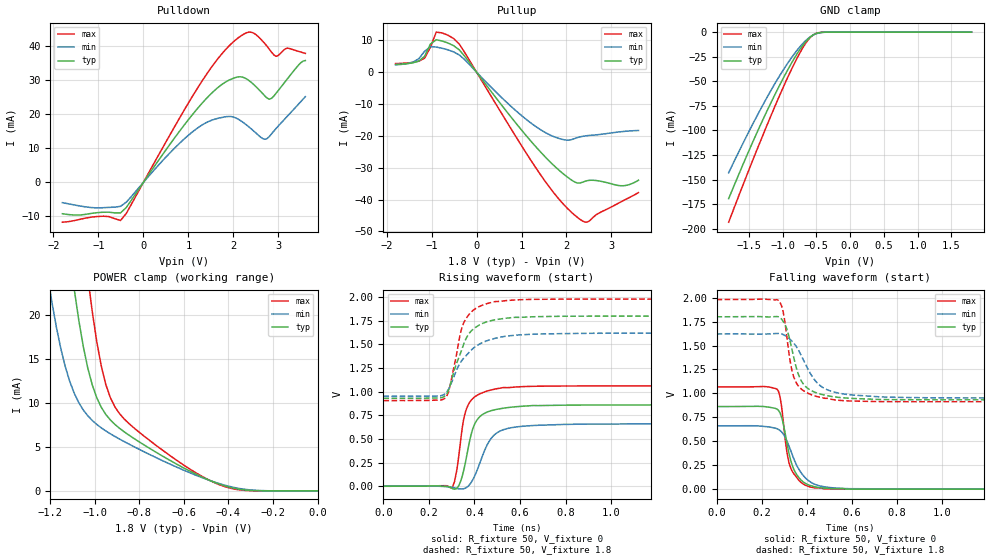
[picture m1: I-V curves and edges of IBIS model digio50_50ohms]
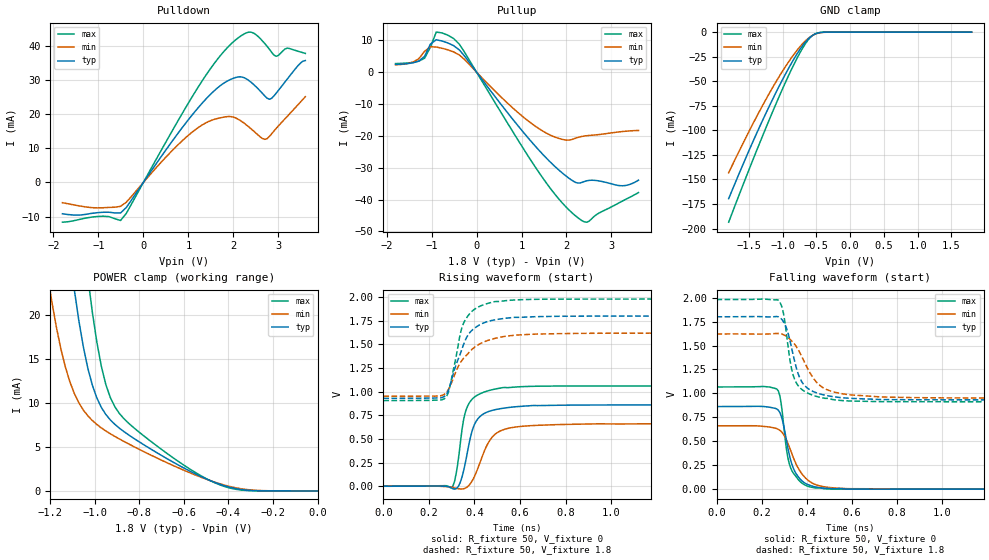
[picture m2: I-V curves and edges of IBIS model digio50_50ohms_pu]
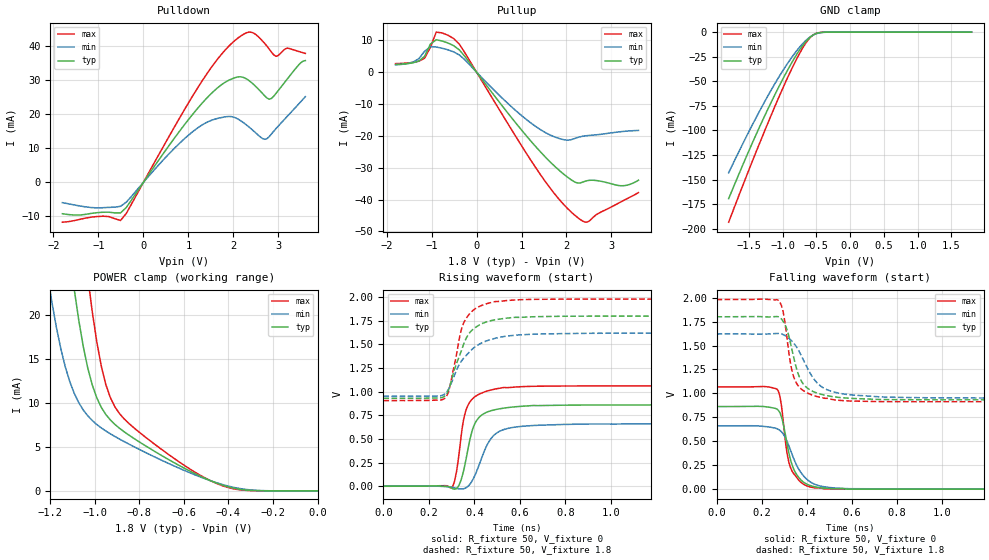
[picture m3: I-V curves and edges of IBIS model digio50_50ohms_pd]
[IBIS ver]   4.0
[File name]   tusb1210.ibs
[File rev]   1.0
[Date]   Thu Nov 25 16:58:20 2010
[Source]   Texas Instruments Incorporated.
   Analog-eLab, HPA
   12500 TI Blvd
   Dallas, TX -75243
   For Support e-mail: elab_ibis@list.ti.com
[Notes] Reision History: 1.0
- Combined Pulldown/Pull up for dn_ls, dn_hs, dn_fs, dp_ls, dp_hs,dp_fs reflects
  the behavior based on simulations.
- GND Clamp value of digio50_50ohms_pu never becomming zero reflects
  the behavior based on simulations.
- POWER Clamp value of digio50_50ohms_pd never becomming zero reflects
  the behavior based on simulations.
[Disclaimer]
 This product is designed as an aid for customers of Texas Instruments.
 No warranties, either expressed or implied, with respect to this third
 party software (if any) or with respect to its fitness for any
 particular purpose is claimed by Texas Instruments or the author. The
 software (if any) is provided solely on an "as is" basis. The entire
 risk as to its quality and performance is with the customer
[Copyright] (C) Copyright 2010 Texas Instruments Incorporated.
   All rights reserved.
|   COMPONENT: TUSB1210
[Component]   TUSB1210
[Manufacturer]   Texas Instruments.
[Package]
|   typ   min   max
R_pkg   6.77e-02  1.30e-03  1.34e-01
L_pkg   1.06e-09  1.42e-10  1.98e-09
C_pkg   1.51e-13  8.64e-14  2.16e-13
[Pin] signal_name   model_name  R_pin   L_pin   C_pin
1   REFCLK   in50_vio_rst0	 1.34e-01  1.98e-09  2.08e-13
2   NXT   digio50_50ohms_ppud 1.17e-01  1.71e-09  2.12e-13
3   DATA0   digio50_50ohms_ppud 1.08e-01  1.56e-09  1.99e-13
4   DATA1   digio50_50ohms_ppud 1.03e-01  1.49e-09  1.93e-13
5   DATA2   digio50_50ohms_ppud 1.03e-01  1.49e-09  1.97e-13
6   DATA3   digio50_50ohms_ppud 1.07e-01  1.56e-09  2.05e-13
7   DATA4   digio50_50ohms_ppud 1.14e-01  1.67e-09  2.05e-13
9   DATA5   digio50_50ohms_ppud 1.30e-03  1.48e-10  8.64e-14
10   DATA6   digio50_50ohms_ppud 1.27e-01  1.87e-09  1.95e-13
11   CS   in50_vio_rst0	 1.08e-01  1.56e-09  1.97e-13
12   NC   NC   1.04e-01  1.50e-09  1.95e-13
13   DATA7   digio50_50ohms_ppud 1.12e-01  1.63e-09  2.03e-13
14   REFSEL2   in50_vio_rst1	 1.13e-01  1.64e-09  2.01e-13
17   CPEN   digout_od_os_3p1	 1.11e-01  1.60e-09  1.95e-13
18   DP   dp   1.30e-03  1.42e-10  1.02e-13
19   DM   dn   1.30e-03  1.48e-10  8.64e-14
20   VDD33   Power		 1.32e-01  1.94e-09  1.99e-13
21   VBAT   Power		 1.23e-01  1.80e-09  2.16e-13
22   VBUS   Power		 1.15e-01  1.67e-09  2.15e-13
23   ID   NC   1.08e-01  1.55e-09  1.99e-13
26   CLOCK   digio50_50ohms_ppud 1.04e-01  1.50e-09  1.91e-13
27   RESETB   in50_vio_rst0	 1.04e-01  1.49e-09  1.90e-13
28   VDD18_1   Power		 1.12e-01  1.62e-09  1.95e-13
29   STP   digio50_50ohms_ppud 1.30e-03  1.48e-10  8.64e-14
30   VDD18_2   Power		 1.30e-03  1.48e-10  8.64e-14
31   DIR   digio50_50ohms_ppud 1.14e-01  1.66e-09  2.01e-13
32   VDDIO   Power		 1.05e-01  1.52e-09  1.95e-13
| Remark: If you runnin LS and FS simulation in differential Rx mode,
|   please uncomment "For LS and FS simulation" line.
|   While for HS Simulation in differential Rx mode,
|   uncomment "For HS simulation only" line. Please do take note only
|   one line can be sitch on for specific simulation.
[Diff Pin] inv_pin vdiff tdelay_typ tdelay_min tdelay_max
|18 19   0.200V   NA   NA   NA   |For LS/FS simulation only
18 19   0.150V   NA   NA   NA   |For HS simulation only
[Model Selector]   digio50_50ohms_ppud
digio50_50ohms   Pullup-down disabled
digio50_50ohms_pu   Pullup enabled
digio50_50ohms_pd   Pulldown enabled
[Model Selector]   digout_od_os_3p1
digout_od_3p1   Open-drain mode
digout_os_3p1   Open-source mode
digout_cmos_3p1   CMOS mode
[Model Selector]   out50_bat
out50_bat_cmos   Output buffer under VBAT NMOS/PMOS enabled
out50_bat_nmos   Output buffer under VBAT NMOS enabled
out50_bat_pmos   Output buffer under VBAT PMOS enabled
[Model Selector]  dp
dp_fs   Full-Speed mode
dp_hs   High-Speed mode
dp_ls   Low-Speed mode
[Model Selector]  dn
dn_fs   Full-Speed mode
dn_hs   High-Speed mode
dn_ls   Low-Speed mode
| Models and submodels in the file (17): digio50_50ohms (I/O), digio50_50ohms_pu (I/O), digio50_50ohms_pd (I/O), in50_vio_rst0 (Input), in50_vio_rst1 (Input), out50_bat_cmos (Output), out50_bat_nmos (Open_drain), out50_bat_pmos (Open_source), dp_fs (I/O), dp_hs (I/O), dp_ls (I/O), dn_fs (I/O), dn_hs (I/O), dn_ls (I/O), digout_cmos_3p1 (Output), digout_od_3p1 (Open_drain), digout_os_3p1 (Open_source)
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|   Model: digio50_50ohms
|   Description:  I/O buffer for ULPI buffer PU/PD disabled
[Model]   digio50_50ohms
Model_type   I/O
Polarity   Non-Inverting
Enable   Active-Low
Vinh =   1.667
Vinl =   1.364
Vmeas =   0.900
Vref =   0
Cref =   5e-12
Rref =   100e3
|variable   typ   min   max
C_comp   1.086p   1.040p   1.121p
[Model Spec]
|Thresholds   typ   min   max
Vinh+   1.667   1.500   1.833
Vinh-   1.364   1.227   1.500
Vinl+   1.667   1.500   1.833
Vinl-   1.364   1.227   1.500
[Temperature Range]   27   125   -40
[Voltage Range]   1.8   1.62   1.98
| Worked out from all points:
|   slope of the pulldown table from 0 to 0.27 V, typ, clamps not added: 51.8 ohm
|   slope of the pullup table from 0 to 0.27 V, typ, clamps not added: 53.2 ohm
|   GND clamp passes 1 mA (typ) near -0.48 V on its own axis
|   POWER clamp passes 1 mA (typ) near -0.47 V on its own axis
|   rising waveform, R_fixture 50, V_fixture 0: 20-80 % time 54.8ps typ, 76.2ps min, 45.4ps max; typ from 0 V to 0.86 V
|   rising waveform, R_fixture 50, V_fixture 1.8: 20-80 % time 82.7ps typ, 112ps min, 63.2ps max; typ from 0.931 V to 1.8 V
|   falling waveform, R_fixture 50, V_fixture 0: 20-80 % time 55.1ps typ, 81.7ps min, 41.4ps max; typ from 0.863 V to 0 V
|   falling waveform, R_fixture 50, V_fixture 1.8: 20-80 % time 65ps typ, 103ps min, 48.7ps max; typ from 1.8 V to 0.932 V
[GND Clamp]
| digio50_50ohms
|Voltage   I(typ)   I(min)   I(max)
-1.8V     -169.5mA   -143.1mA   -193.4mA
-1.598V   -136.3mA   -114.5mA   -157.3mA
-1.395V   -104.5mA   -87.3mA    -122.2mA
-1.193V   -74.69mA   -61.74mA   -88.34mA
-1.032V   -52.26mA   -42.95mA   -62.34mA
-869.7mV  -31.66mA   -26.14mA   -38mA
-748.3mV  -18.08mA   -15.27mA   -21.59mA
-627mV    -7.357mA   -6.7mA     -8.334mA
-546.1mV  -2.821mA   -2.927mA   -2.841mA
-465.2mV  -709.6uA   -933.8uA   -580uA
-303.4mV  -9.124uA   -34.65uA   -2.526uA
1.8V      19.41nA    6.754uA    15.04nA
[POWER Clamp]
| digio50_50ohms
|Voltage   I(typ)   I(min)   I(max)
-1.8V     230mA      184.4mA    260.1mA
-1.214V   50.81mA    24.76mA    72.72mA
-1.193V   45.55mA    21.5mA     66.74mA
-1.153V   35.62mA    16.15mA    55.07mA
-1.092V   22.81mA    11.06mA    38.57mA
-1.032V   13.92mA    8.517mA    24.25mA
-1.011V   12mA       7.982mA    20.28mA
-991mV    10.55mA    7.534mA    16.89mA
-930.3mV  8.051mA    6.48mA     10.58mA
-829.2mV  6.029mA    5.081mA    7.251mA
-424.7mV  636.6uA    708.5uA    557.6uA
0V        19.41nA    47.88nA    41nA
[Pulldown]
| digio50_50ohms
|Voltage   I(typ)   I(min)   I(max)
-1.8V     -9.222mA   -5.96mA    -11.7mA
-895.8mV  -8.773mA   -7.446mA   -9.946mA
-508.3mV  -8.983mA   -7.037mA   -11.2mA
1.2V      21.68mA    15.95mA    27.64mA
1.8V      29.29mA    19.23mA    38.64mA
2.15V     31.05mA    18.24mA    42.9mA
2.45V     28.8mA     15.11mA    43.89mA
2.65V     26.12mA    12.89mA    41.53mA
2.8V      24.46mA    13.51mA    39.15mA
2.95V     26.21mA    15.86mA    37.06mA
3.2V      30.42mA    19.45mA    39.49mA
3.6V      35.82mA    25.21mA    37.92mA
[Pullup]
| digio50_50ohms
|Voltage   I(typ)   I(min)   I(max)
-1.8V     2.414mA    2.279mA    2.667mA
-1.413V   2.907mA    3.119mA    3.042mA
-1.154V   4.963mA    6.516mA    4.36mA
-1.025V   8.782mA    7.956mA    7.803mA
-895.8mV  10.15mA    7.861mA    12.55mA
-508.3mV  8.286mA    6.333mA    10.52mA
1.4V      -24.71mA   -17.87mA   -31.75mA
1.95V     -32.18mA   -21.25mA   -41.74mA
2.35V     -34.6mA    -20.18mA   -46.68mA
2.5V      -33.98mA   -19.9mA    -46.81mA
3.25V     -35.67mA   -18.66mA   -40.43mA
3.6V      -33.93mA   -18.33mA   -37.83mA
[Ramp]
| digio50_50ohms
|variable   typ   min   max
dV/dt_r   0.863/5.506e-11   0.661/7.618e-11   1.068/4.610e-11
dV/dt_f   0.870/6.539e-11   0.669/1.029e-10   1.074/4.951e-11
R_load =   50
[Rising Waveform]
| digio50_50ohms
R_fixture =   50
V_fixture =   0
V_fixture_min =   0
V_fixture_max =   0
|Time   V(typ)   V(min)   V(max)
0s        348.4uV    407.9uV    39.07nV
303.5ps   -25.21mV   -11.62mV   -7.697mV
321.2ps   -23.49mV   -23.4mV    153.7mV
341.4ps   67.66mV    -28.79mV   526.8mV
356.6ps   210mV      -23.23mV   751.6mV
381.4ps   507.3mV    25.8mV     896.4mV
414.2ps   710.8mV    185.8mV    965.6mV
480.6ps   804mV      527.1mV    1.023V
604.6ps   845.1mV    632.9mV    1.053V
9.107ns   860.3mV    661.1mV    1.062V
[Rising Waveform]
| digio50_50ohms
R_fixture =   50
V_fixture =   1.8
V_fixture_min =   1.62
V_fixture_max =   1.98
|Time   V(typ)   V(min)   V(max)
0s        930.6mV    951.8mV    906.4mV
268ps     950.3mV    973.3mV    926mV
285.7ps   1.014V     1.024V     994.6mV
294.6ps   1.081V     1.067V     1.082V
312.3ps   1.237V     1.175V     1.287V
341.4ps   1.426V     1.319V     1.648V
370.8ps   1.596V     1.401V     1.8V
445.2ps   1.732V     1.53V      1.924V
586.9ps   1.787V     1.599V     1.972V
9.107ns   1.8V       1.62V      1.98V
[Falling Waveform]
| digio50_50ohms
R_fixture =   50
V_fixture =   0
V_fixture_min =   0
V_fixture_max =   0
|Time   V(typ)   V(min)   V(max)
0s        862.7mV    661.7mV    1.067V
267.2ps   837.3mV    631.9mV    1.046V
281.1ps   798.7mV    614mV      971.1mV
295.9ps   682.3mV    575mV      707.6mV
311.7ps   487.1mV    504mV      392.5mV
333.3ps   266.7mV    374.7mV    197.4mV
358.7ps   141.4mV    234.5mV    111.7mV
398.7ps   54.93mV    107.4mV    36.34mV
488.6ps   8.651mV    21.17mV    2.83mV
10.37ns   31.52uV    30.23uV    11.42uV
[Falling Waveform]
| digio50_50ohms
R_fixture =   50
V_fixture =   1.8
V_fixture_min =   1.62
V_fixture_max =   1.98
|Time   V(typ)   V(min)   V(max)
0s        1.8V       1.621V     1.98V
274.2ps   1.8V       1.625V     1.973V
295.9ps   1.751V     1.614V     1.846V
311.7ps   1.671V     1.592V     1.591V
333.3ps   1.471V     1.548V     1.251V
361.8ps   1.207V     1.458V     1.081V
394ps     1.073V     1.306V     1.016V
454ps     997.5mV    1.092V     961.6mV
592.3ps   948.2mV    984.8mV    920.5mV
10.37ns   932.4mV    951.5mV    912.2mV
|   Model: digio50_50ohms_pu
|   Description:  I/O buffer for ULPI buffer PU enabled
[Model]   digio50_50ohms_pu
Model_type   I/O
Polarity   Non-Inverting
Enable   Active-Low
Vinh =   1.667
Vinl =   1.364
Vmeas =   0.900
Vref =   0
Cref =   5e-12
Rref =   100e3
|variable   typ   min   max
C_comp   1.086p   1.040p   1.121p
[Model Spec]
|Thresholds   typ   min   max
Vinh+   1.667   1.500   1.833
Vinh-   1.364   1.227   1.500
Vinl+   1.667   1.500   1.833
Vinl-   1.364   1.227   1.500
[Temperature Range]   27   125   -40
[Voltage Range]   1.8   1.62   1.98
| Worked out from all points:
|   slope of the pulldown table from 0 to 0.27 V, typ, clamps not added: 51.8 ohm
|   slope of the pullup table from 0 to 0.27 V, typ, clamps not added: 53.3 ohm
|   GND clamp passes 1 mA (typ) near -0.48 V on its own axis
|   POWER clamp passes 1 mA (typ) near -0.46 V on its own axis
|   rising waveform, R_fixture 50, V_fixture 0: 20-80 % time 54.8ps typ, 76.2ps min, 45.4ps max; typ from 0 V to 0.86 V
|   rising waveform, R_fixture 50, V_fixture 1.8: 20-80 % time 82.7ps typ, 112ps min, 63.2ps max; typ from 0.931 V to 1.8 V
|   falling waveform, R_fixture 50, V_fixture 0: 20-80 % time 55.1ps typ, 81.7ps min, 41.4ps max; typ from 0.863 V to 0 V
|   falling waveform, R_fixture 50, V_fixture 1.8: 20-80 % time 65ps typ, 103ps min, 48.7ps max; typ from 1.8 V to 0.932 V
[GND Clamp]
| digio50_50ohms_pu
|Voltage   I(typ)   I(min)   I(max)
-1.8V     -169.5mA   -143.1mA   -193.5mA
-1.598V   -136.3mA   -114.6mA   -157.3mA
-1.395V   -104.6mA   -87.32mA   -122.3mA
-1.193V   -74.72mA   -61.76mA   -88.37mA
-1.032V   -52.29mA   -42.97mA   -62.37mA
-869.7mV  -31.68mA   -26.16mA   -38.03mA
-748.3mV  -18.1mA    -15.28mA   -21.62mA
-627mV    -7.378mA   -6.717mA   -8.361mA
-546.1mV  -2.842mA   -2.944mA   -2.868mA
-465.2mV  -730.7uA   -950.8uA   -606.8uA
-303.4mV  -29.85uA   -51.32uA   -28.89uA
1.8V      19.33nA    7.928uA    -2.076uA
[POWER Clamp]
| digio50_50ohms_pu
|Voltage   I(typ)   I(min)   I(max)
-1.8V     230mA      184.4mA    260.1mA
-1.214V   50.81mA    24.76mA    72.72mA
-1.193V   45.55mA    21.5mA     66.74mA
-1.153V   35.62mA    16.15mA    55.07mA
-1.092V   22.81mA    11.06mA    38.57mA
-1.032V   13.92mA    8.519mA    24.25mA
-1.011V   12mA       7.984mA    20.29mA
-991mV    10.55mA    7.536mA    16.89mA
-930.3mV  8.053mA    6.482mA    10.58mA
-829.2mV  6.032mA    5.083mA    7.254mA
-424.7mV  638.9uA    710.2uA    560.6uA
0V        19.33nA    47.31nA    40.57nA
[Pulldown]
| digio50_50ohms_pu
|Voltage   I(typ)   I(min)   I(max)
-1.8V     -9.196mA   -5.938mA   -11.67mA
-895.8mV  -8.751mA   -7.428mA   -9.918mA
-508.3mV  -8.962mA   -7.02mA    -11.17mA
1.2V      21.68mA    15.95mA    27.65mA
1.8V      29.29mA    19.23mA    38.65mA
2.15V     31.05mA    18.23mA    42.9mA
2.45V     28.79mA    15.11mA    43.88mA
2.65V     26.12mA    12.89mA    41.52mA
2.8V      24.46mA    13.5mA     39.14mA
2.95V     26.2mA     15.86mA    37.06mA
3.2V      30.42mA    19.45mA    39.49mA
3.6V      35.82mA    25.21mA    37.92mA
[Pullup]
| digio50_50ohms_pu
|Voltage   I(typ)   I(min)   I(max)
-1.8V     2.413mA    2.278mA    2.666mA
-1.413V   2.906mA    3.118mA    3.042mA
-1.154V   4.962mA    6.515mA    4.359mA
-1.025V   8.78mA     7.954mA    7.801mA
-895.8mV  10.15mA    7.859mA    12.55mA
-508.3mV  8.284mA    6.332mA    10.52mA
1.4V      -24.69mA   -17.86mA   -31.73mA
1.95V     -32.16mA   -21.24mA   -41.72mA
2.35V     -34.57mA   -20.16mA   -46.65mA
2.5V      -33.96mA   -19.88mA   -46.78mA
3.25V     -35.65mA   -18.63mA   -40.4mA
3.6V      -33.9mA    -18.31mA   -37.8mA
[Ramp]
| digio50_50ohms_pu
|variable   typ   min   max
dV/dt_r   0.863/5.506e-11   0.661/7.618e-11   1.068/4.610e-11
dV/dt_f   0.870/6.539e-11   0.669/1.029e-10   1.074/4.951e-11
R_load =   50
[Rising Waveform]
| digio50_50ohms_pu
R_fixture =   50
V_fixture =   0
V_fixture_min =   0
V_fixture_max =   0
|Time   V(typ)   V(min)   V(max)
0s        348.5uV    407.9uV    39.08nV
303.5ps   -25.3mV    -11.66mV   -7.449mV
321.2ps   -23.38mV   -23.43mV   154.7mV
336.4ps   34.32mV    -28.24mV   425.4mV
351.6ps   156.8mV    -26.57mV   696.2mV
374.4ps   427.1mV    5.616mV    869.1mV
418.6ps   723.7mV    213.9mV    971.3mV
471.8ps   798.1mV    501.1mV    1.018V
524.9ps   824.7mV    596.3mV    1.044V
7.289ns   860.3mV    661.1mV    1.062V
[Rising Waveform]
| digio50_50ohms_pu
R_fixture =   50
V_fixture =   1.8
V_fixture_min =   1.62
V_fixture_max =   1.98
|Time   V(typ)   V(min)   V(max)
0s        930.6mV    951.8mV    906.4mV
268.1ps   950.5mV    973.5mV    926.2mV
285.8ps   1.015V     1.024V     995.2mV
294.7ps   1.082V     1.068V     1.083V
312.4ps   1.238V     1.175V     1.288V
341.5ps   1.426V     1.319V     1.649V
367.3ps   1.581V     1.392V     1.788V
439.3ps   1.726V     1.524V     1.919V
569.2ps   1.786V     1.595V     1.969V
7.289ns   1.8V       1.62V      1.98V
[Falling Waveform]
| digio50_50ohms_pu
R_fixture =   50
V_fixture =   0
V_fixture_min =   0
V_fixture_max =   0
|Time   V(typ)   V(min)   V(max)
0s        862.7mV    661.7mV    1.067V
267.2ps   837.4mV    632mV      1.046V
281ps     799.2mV    614.2mV    972.1mV
295.8ps   683.3mV    575.3mV    709.5mV
311.6ps   488.2mV    504.4mV    393.7mV
333.2ps   267.2mV    375.1mV    197.7mV
358.6ps   141.6mV    234.8mV    111.9mV
398.6ps   54.98mV    107.5mV    36.37mV
488.6ps   8.649mV    21.16mV    2.828mV
10.37ns   31.5uV     30.21uV    11.41uV
[Falling Waveform]
| digio50_50ohms_pu
R_fixture =   50
V_fixture =   1.8
V_fixture_min =   1.62
V_fixture_max =   1.98
|Time   V(typ)   V(min)   V(max)
0s        1.8V       1.621V     1.98V
274.1ps   1.8V       1.625V     1.973V
295.8ps   1.752V     1.614V     1.847V
311.6ps   1.672V     1.593V     1.593V
333.2ps   1.472V     1.548V     1.252V
361.7ps   1.207V     1.458V     1.081V
394ps     1.073V     1.306V     1.016V
454ps     997.5mV    1.092V     961.6mV
592.4ps   948.2mV    984.8mV    920.4mV
10.37ns   932.4mV    951.5mV    912.2mV
|   Model: digio50_50ohms_pd
|   Description:  I/O buffer for ULPI buffer PD enabled
[Model]   digio50_50ohms_pd
Model_type   I/O
Polarity   Non-Inverting
Enable   Active-Low
Vinh =   1.667
Vinl =   1.364
Vmeas =   0.900
Vref =   0
Cref =   5e-12
Rref =   100e3
|variable   typ   min   max
C_comp   1.086p   1.040p   1.121p
[Model Spec]
|Thresholds   typ   min   max
Vinh+   1.667   1.500   1.833
Vinh-   1.364   1.227   1.500
Vinl+   1.667   1.500   1.833
Vinl-   1.364   1.227   1.500
[Temperature Range]   27   125   -40
[Voltage Range]   1.8   1.62   1.98
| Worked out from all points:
|   slope of the pulldown table from 0 to 0.27 V, typ, clamps not added: 51.8 ohm
|   slope of the pullup table from 0 to 0.27 V, typ, clamps not added: 53.3 ohm
|   GND clamp passes 1 mA (typ) near -0.48 V on its own axis
|   POWER clamp passes 1 mA (typ) near -0.46 V on its own axis
|   rising waveform, R_fixture 50, V_fixture 0: 20-80 % time 54.8ps typ, 76.2ps min, 45.4ps max; typ from 0 V to 0.86 V
|   rising waveform, R_fixture 50, V_fixture 1.8: 20-80 % time 82.7ps typ, 112ps min, 63.2ps max; typ from 0.931 V to 1.8 V
|   falling waveform, R_fixture 50, V_fixture 0: 20-80 % time 55.1ps typ, 81.7ps min, 41.4ps max; typ from 0.863 V to 0 V
|   falling waveform, R_fixture 50, V_fixture 1.8: 20-80 % time 65ps typ, 103ps min, 48.7ps max; typ from 1.8 V to 0.932 V
[GND Clamp]
| digio50_50ohms_pd
|Voltage   I(typ)   I(min)   I(max)
-1.8V     -169.5mA   -143.1mA   -193.4mA
-1.598V   -136.3mA   -114.6mA   -157.3mA
-1.395V   -104.5mA   -87.3mA    -122.2mA
-1.193V   -74.69mA   -61.74mA   -88.35mA
-1.032V   -52.27mA   -42.95mA   -62.34mA
-869.7mV  -31.66mA   -26.14mA   -38mA
-748.3mV  -18.09mA   -15.27mA   -21.6mA
-627mV    -7.36mA    -6.702mA   -8.338mA
-546.1mV  -2.824mA   -2.929mA   -2.845mA
-465.2mV  -712.7uA   -936.2uA   -583.8uA
-303.4mV  -11.86uA   -36.83uA   -5.896uA
1.8V      18.01uA    22.42uA    20.92uA
[POWER Clamp]
| digio50_50ohms_pd
|Voltage   I(typ)   I(min)   I(max)
-1.8V     230mA      184.4mA    260.2mA
-1.214V   50.83mA    24.78mA    72.75mA
-1.193V   45.58mA    21.52mA    66.77mA
-1.153V   35.64mA    16.17mA    55.09mA
-1.092V   22.84mA    11.07mA    38.6mA
-1.032V   13.94mA    8.534mA    24.28mA
-1.011V   12.02mA    7.999mA    20.31mA
-991mV    10.57mA    7.551mA    16.91mA
-930.3mV  8.072mA    6.496mA    10.61mA
-829.2mV  6.05mA     5.098mA    7.277mA
-424.7mV  656.8uA    724.7uA    583.6uA
0V        18.01uA    14.54uA    23.03uA
[Pulldown]
| digio50_50ohms_pd
|Voltage   I(typ)   I(min)   I(max)
-1.8V     -9.22mA    -5.958mA   -11.7mA
-895.8mV  -8.77mA    -7.444mA   -9.943mA
-508.3mV  -8.98mA    -7.035mA   -11.2mA
1.2V      21.66mA    15.94mA    27.63mA
1.8V      29.27mA    19.22mA    38.62mA
2.15V     31.03mA    18.22mA    42.88mA
2.45V     28.78mA    15.1mA     43.86mA
2.65V     26.1mA     12.87mA    41.5mA
2.8V      24.44mA    13.49mA    39.12mA
2.95V     26.18mA    15.84mA    37.03mA
3.2V      30.4mA     19.43mA    39.46mA
3.6V      35.79mA    25.19mA    37.89mA
[Pullup]
| digio50_50ohms_pd
|Voltage   I(typ)   I(min)   I(max)
-1.8V     2.387mA    2.256mA    2.633mA
-1.413V   2.882mA    3.098mA    3.012mA
-1.154V   4.94mA     6.499mA    4.331mA
-1.025V   8.76mA     7.94mA     7.775mA
-895.8mV  10.13mA    7.845mA    12.53mA
-508.3mV  8.266mA    6.317mA    10.5mA
1.4V      -24.71mA   -17.87mA   -31.75mA
1.95V     -32.18mA   -21.25mA   -41.74mA
2.35V     -34.59mA   -20.17mA   -46.67mA
2.5V      -33.98mA   -19.89mA   -46.81mA
3.25V     -35.67mA   -18.65mA   -40.43mA
3.6V      -33.93mA   -18.33mA   -37.83mA
[Ramp]
| digio50_50ohms_pd
|variable   typ   min   max
dV/dt_r   0.863/5.506e-11   0.661/7.618e-11   1.068/4.610e-11
dV/dt_f   0.870/6.539e-11   0.669/1.029e-10   1.074/4.951e-11
R_load =   50
[Rising Waveform]
| digio50_50ohms_pd
R_fixture =   50
V_fixture =   0
V_fixture_min =   0
V_fixture_max =   0
|Time   V(typ)   V(min)   V(max)
0s        348.5uV    407.9uV    39.08nV
303.5ps   -25.2mV    -11.62mV   -7.722mV
321.2ps   -23.49mV   -23.4mV    153.8mV
336.4ps   34.04mV    -28.23mV   424.5mV
356.6ps   210.2mV    -23.21mV   751.8mV
377.9ps   468.9mV    15.1mV     883.7mV
414.2ps   711mV      186.2mV    965.6mV
480.7ps   804.1mV    527.4mV    1.023V
595.9ps   843.6mV    630.8mV    1.052V
9.11ns    860.3mV    661.1mV    1.062V
[Rising Waveform]
| digio50_50ohms_pd
R_fixture =   50
V_fixture =   1.8
V_fixture_min =   1.62
V_fixture_max =   1.98
|Time   V(typ)   V(min)   V(max)
0s        930.6mV    951.8mV    906.4mV
268ps     950.3mV    973.3mV    926mV
285.7ps   1.014V     1.024V     994.5mV
294.6ps   1.081V     1.067V     1.081V
312.3ps   1.237V     1.175V     1.287V
341.4ps   1.426V     1.319V     1.648V
370.8ps   1.596V     1.401V     1.8V
445.3ps   1.732V     1.53V      1.924V
587.1ps   1.787V     1.599V     1.972V
9.11ns    1.8V       1.62V      1.98V
[Falling Waveform]
| digio50_50ohms_pd
R_fixture =   50
V_fixture =   0
V_fixture_min =   0
V_fixture_max =   0
|Time   V(typ)   V(min)   V(max)
0s        862.7mV    661.7mV    1.067V
267.2ps   837.4mV    632mV      1.046V
281ps     799.1mV    614.1mV    972mV
295.8ps   683mV      575.2mV    709mV
311.7ps   487.7mV    504.2mV    393.2mV
333.3ps   266.9mV    374.9mV    197.5mV
358.7ps   141.4mV    234.5mV    111.7mV
398.7ps   54.88mV    107.3mV    36.3mV
488.7ps   8.631mV    21.12mV    2.814mV
10.37ns   31.52uV    30.23uV    11.43uV
[Falling Waveform]
| digio50_50ohms_pd
R_fixture =   50
V_fixture =   1.8
V_fixture_min =   1.62
V_fixture_max =   1.98
|Time   V(typ)   V(min)   V(max)
0s        1.8V       1.621V     1.98V
274.1ps   1.8V       1.625V     1.973V
295.8ps   1.752V     1.614V     1.846V
311.7ps   1.671V     1.593V     1.592V
333.3ps   1.471V     1.548V     1.252V
361.8ps   1.207V     1.458V     1.081V
394.1ps   1.073V     1.306V     1.016V
454.1ps   997.4mV    1.092V     961.6mV
592.6ps   948.2mV    984.7mV    920.4mV
10.37ns   932.4mV    951.5mV    912.2mV
